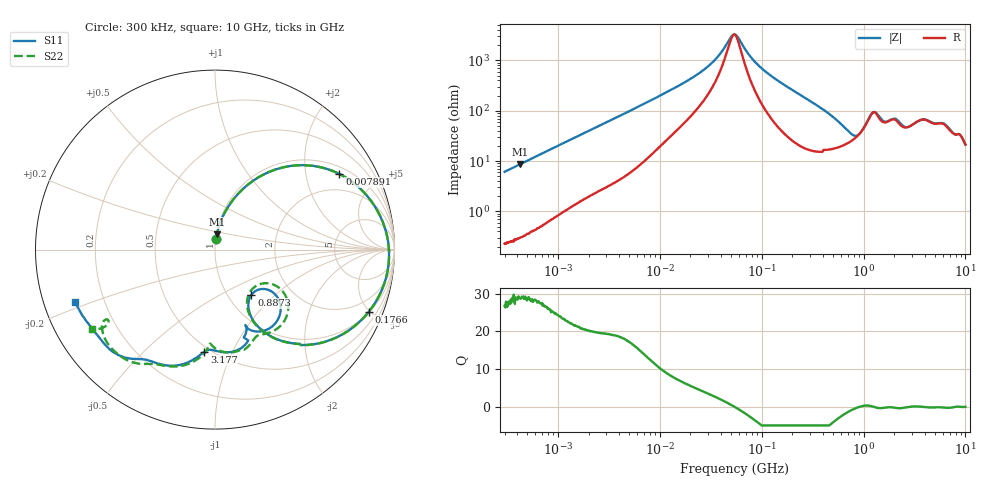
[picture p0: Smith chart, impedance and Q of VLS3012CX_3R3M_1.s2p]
! S-Parameter Data Generated by TDK Corporation
! Copyright(C) 2020 TDK Corporation.
! All Rights Reserved.
! TDK P/N: VLS3012CX-3R3M-1 (Inductor)
! Property: L=3.3uH at 1MHz
! Size(LxWxT): 3x3x1.2mm
! Model Type: s2p (Touchstone File Format Version 1.0)
! Frequency: DC=Yes Start=0.3MHz Stop=10000MHz 802points Log-sweep
! Model Generated on Aug. 18, 2020
! Port Assignments:
!  1 ---@@@--- 2
! Applicable Conditions:
!  Temperature = 25 degC
!  DC Bias Current = 0 A
!  Small Signal Operation
! Terms and conditions regarding TDK Simulation Models
! (1)This simulation model is being provided solely for informational purposes. Please refer to the specifications of the products in terms of detailed characteristics of such products.
! (2)In no event shall TDK Corporation of any of its subsidiaries be liable for any loss or damage arising, directly or indirectly,
!  From any information contained in this simulation model, including, but not limited to loss or damages arising from any inaccuracies, omissions or errors in connection with such information.
! (3)Any and all copyrights on this simulation model are owned by TDK Corporation.
!  Duplication or redistribution of this simulation model without prior written permission from TDK Corporation is prohibited.
! (4)This simulation model is subject to any modification or change without any prior notice.
! (5)Neither TDK Corporation nor any of its subsidiaries shall make any warranty, express or implied,
!  Including but not limited to the correctness, implied warranties of merchantability and fitness for a particular purpose with respect to this simulation models.
! (6)The use of this simulation model shall be deemed to have consented to the terms and conditions hereof.
# Hz S MA R 50
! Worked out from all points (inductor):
!   801 points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, 300 kHz to 10 GHz, reference 50 ohm
!   read as one part in series: L = 3.24 uH near 318.3 kHz
!   highest Q = 28.9 at 421.7 kHz (marker M1), where L = 3.24 uH
!   self-resonance near 53.74 MHz
!   S11 on the Smith chart (normalised r, x): 300 kHz: 1.00, +0.12; 7.891 MHz: 1.26, +3.10; 176.6 MHz: 1.03, -4.91; 887.3 MHz: 1.28, -0.72; 3.177 GHz: 0.46, -0.79; 10 GHz: 0.10, -0.18
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300000  0.06108 84.3  0.9959 -3.5  0.9959 -3.5  0.06079 84.4
421743  0.08516 83.0  0.9934 -4.9  0.9934 -4.9  0.08507 83.2
1713600  0.3172 68.7  0.9332 -18.5  0.9331 -18.5  0.3173 68.7
4053600  0.604 49.7  0.765 -37.2  0.7649 -37.2  0.604 49.7
7890546  0.8114 31.3  0.5237 -54.2  0.5237 -54.2  0.8114 31.3
9671944  0.8536 26.1  0.4464 -58.5  0.4463 -58.4  0.8535 26.1
2.725275e7  0.9539 7.3  0.1451 -68.3  0.1451 -68.3  0.9539 7.3
5.477226e7  0.9704 -1.7  0.02975 5.7  0.02975 5.7  0.9704 -1.7
9.209736e7  0.9662 -9.1  0.1185 67.7  0.1185 67.6  0.9662 -9.1
1.765741e8  0.9238 -22.1  0.2999 62.0  0.2999 62.0  0.9237 -22.2
3.126428e8  0.8052 -39.3  0.516 44.7  0.5159 44.7  0.8049 -39.4
5.105874e8  0.5937 -56.1  0.6892 21.8  0.6892 21.8  0.5918 -56.4
8.872678e8  0.3236 -51.2  0.7293 -12.5  0.7293 -12.5  0.3068 -50.7
1.069912e9  0.3843 -36.6  0.6225 -25.5  0.6226 -25.5  0.3639 -31.5
1.24442e9  0.5146 -45.6  0.4874 -24.5  0.4875 -24.5  0.5179 -38.0
1.767019e9  0.4576 -67.9  0.5409 -29.1  0.5409 -29.1  0.5423 -66.1
2.264206e9  0.5767 -79.7  0.5175 -31.4  0.5174 -31.4  0.5712 -85.5
3.177248e9  0.5726 -95.9  0.4773 -55.3  0.477 -55.3  0.5564 -94.5
4.166115e9  0.6828 -108.8  0.3627 -63.5  0.3625 -63.5  0.6825 -107.6
6.333834e9  0.785 -130.1  0.276 -78.3  0.2759 -78.2  0.7834 -127.5
8.211115e9  0.8102 -143.8  0.2349 -88.8  0.2351 -88.8  0.7274 -147.4
1e10  0.8303 -159.6  0.2224 -89.5  0.2224 -89.5  0.815 -147.1
